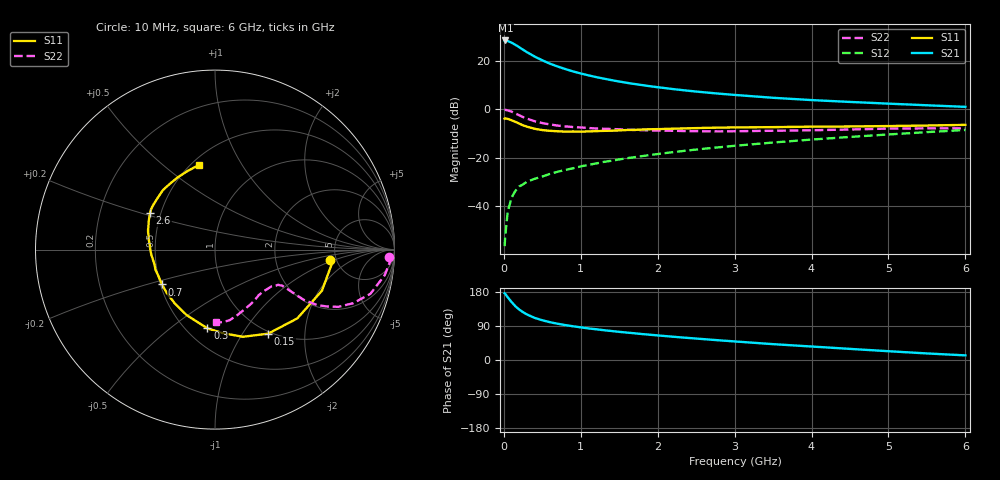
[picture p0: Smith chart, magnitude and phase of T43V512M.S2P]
! Infineon Technologies  Discrete & RF Semiconductors
! BFR182T
! Si NPN RF Bipolar Junction Transistor in SC75
! VCE = 3.5 V  IC = 12 mA
! Common Emitter S-Parameters:  October  1999
# GHz  S  MA  R  50
!  f  S11  S21  S12  S22
! GHz  MAG  ANG  MAG  ANG  MAG  ANG  MAG  ANG
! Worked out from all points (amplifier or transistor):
!   36 points, 10 MHz to 6 GHz, reference 50 ohm
!   highest |S21| = 28.5 dB at 20 MHz (marker M1)
!   |S21| within 3 dB of that: start of sweep to 210.1 MHz
!   unconditionally stable (mu >= 1): 892.2 MHz to 3.745 GHz
!   at 250 MHz: K = 0.50, MSG = 27.8 dB, |S12| = -30.9 dB
!   at 1.4 GHz: K = 1.08, MAG = 14.9 dB, |S12| = -21.2 dB
!   at 6 GHz: K = 0.85, MSG = 4.8 dB, |S12| = -8.5 dB
!   S11 on the Smith chart (normalised r, x): 10 MHz: 4.44, -0.89; 150 MHz: 0.97, -1.31; 300 MHz: 0.63, -0.69; 700 MHz: 0.51, -0.23; 2.6 GHz: 0.44, +0.21; 6 GHz: 0.55, +0.67
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0.01  0.6445 -5.2  26.45 176.0  0.0015 75.0  0.9698 -2.4
0.02  0.6548 -7.3  26.54 174.3  0.0026 86.2  0.9801 -3.5
0.05  0.6384 -21.0  25.86 165.6  0.0076 89.6  0.9561 -8.6
0.1  0.5976 -39.9  23.9 153.1  0.015 74.6  0.9 -15.9
0.15  0.5541 -57.7  21.58 141.9  0.0208 66.2  0.8258 -21.2
0.2  0.5101 -72.2  19.26 133.1  0.0256 64.9  0.7575 -24.9
0.25  0.469 -84.2  17.07 126.1  0.0284 61.3  0.6943 -27.1
0.3  0.4408 -95.5  15.23 120.2  0.032 60.3  0.6467 -28.5
0.4  0.3978 -113.4  12.37 111.2  0.0369 59.6  0.5697 -29.5
0.5  0.3744 -126.8  10.32 104.9  0.0411 59.9  0.5231 -29.2
0.6  0.3613 -137.9  8.794 99.7  0.0467 61.6  0.489 -28.9
0.7  0.3535 -146.7  7.68 95.7  0.0516 62.3  0.4641 -28.6
0.9  0.3501 -161.3  6.087 89.0  0.0609 64.7  0.4321 -28.3
1.1  0.351 -171.8  5.053 83.3  0.0716 65.8  0.4131 -28.8
1.3  0.3608 179.9  4.321 78.6  0.0825 66.6  0.3979 -29.8
1.6  0.3755 170.3  3.54 72.3  0.0983 67.3  0.3818 -32.0
2.2  0.4002 157.6  2.629 61.4  0.1312 67.5  0.3617 -38.4
2.6  0.415 150.7  2.257 55.0  0.1542 67.1  0.3536 -43.5
3.5  0.4307 137.5  1.738 41.8  0.2071 64.1  0.3626 -56.0
4.5  0.4441 124.8  1.427 29.3  0.2703 59.4  0.3851 -71.0
5.5  0.4648 108.6  1.217 17.3  0.3398 53.8  0.4067 -83.8
6  0.4796 100.8  1.13 12.2  0.376 50.1  0.406 -89.1
